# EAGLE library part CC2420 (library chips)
2.4 GHz IEEE 802.15.4 / ZigBee-ready RF Transceiver
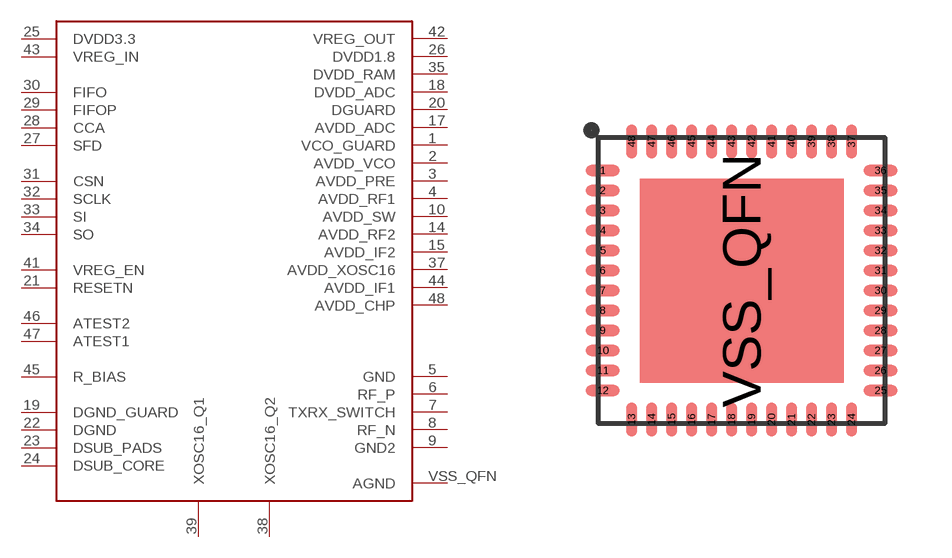
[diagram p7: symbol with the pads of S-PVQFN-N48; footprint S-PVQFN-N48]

Designator prefix U

## CC2420RGZ (DIGIKEY: 296-19585-1-ND)  [S-PVQFN-N48]
1  VCO_GUARD
2  AVDD_VCO
3  AVDD_PRE
4  AVDD_RF1
5  GND
6  RF_P
7  TXRX_SWITCH
8  RF_N
9  GND2
10  AVDD_SW
14  AVDD_RF2
15  AVDD_IF2
17  AVDD_ADC
18  DVDD_ADC
19  DGND_GUARD
20  DGUARD
21  RESETN
22  DGND
23  DSUB_PADS
24  DSUB_CORE
25  DVDD3.3
26  DVDD1.8
27  SFD
28  CCA
29  FIFOP
30  FIFO
31  CSN
32  SCLK
33  SI
34  SO
35  DVDD_RAM
37  AVDD_XOSC16
38  XOSC16_Q2
39  XOSC16_Q1
41  VREG_EN
42  VREG_OUT
43  VREG_IN
44  AVDD_IF1
45  R_BIAS
46  ATEST2
47  ATEST1
48  AVDD_CHP
VSS_QFN  AGND

## Footprint S-PVQFN-N48 (pad centres in mm)
TI RGZ Package
smd 0.85 x 0.28: 1 -3.475,2.75; 2 -3.475,2.25; 3 -3.475,1.75; 4 -3.475,1.25; 5 -3.475,0.75; 6 -3.475,0.25; 7 -3.475,-0.25; 8 -3.475,-0.75; 9 -3.475,-1.25; 10 -3.475,-1.75; 11 -3.475,-2.25; 12 -3.475,-2.75; 25 3.475,-2.75; 26 3.475,-2.25; 27 3.475,-1.75; 28 3.475,-1.25; 29 3.475,-0.75; 30 3.475,-0.25; 31 3.475,0.25; 32 3.475,0.75; 33 3.475,1.25; 34 3.475,1.75; 35 3.475,2.25; 36 3.475,2.75
smd 0.28 x 0.85: 13 -2.75,-3.475; 14 -2.25,-3.475; 15 -1.75,-3.475; 16 -1.25,-3.475; 17 -0.75,-3.475; 18 -0.25,-3.475; 19 0.25,-3.475; 20 0.75,-3.475; 21 1.25,-3.475; 22 1.75,-3.475; 23 2.25,-3.475; 24 2.75,-3.475; 37 2.75,3.475; 38 2.25,3.475; 39 1.75,3.475; 40 1.25,3.475; 41 0.75,3.475; 42 0.25,3.475; 43 -0.25,3.475; 44 -0.75,3.475; 45 -1.25,3.475; 46 -1.75,3.475; 47 -2.25,3.475; 48 -2.75,3.475
smd 5.1 x 5.1: VSS_QFN 0,0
